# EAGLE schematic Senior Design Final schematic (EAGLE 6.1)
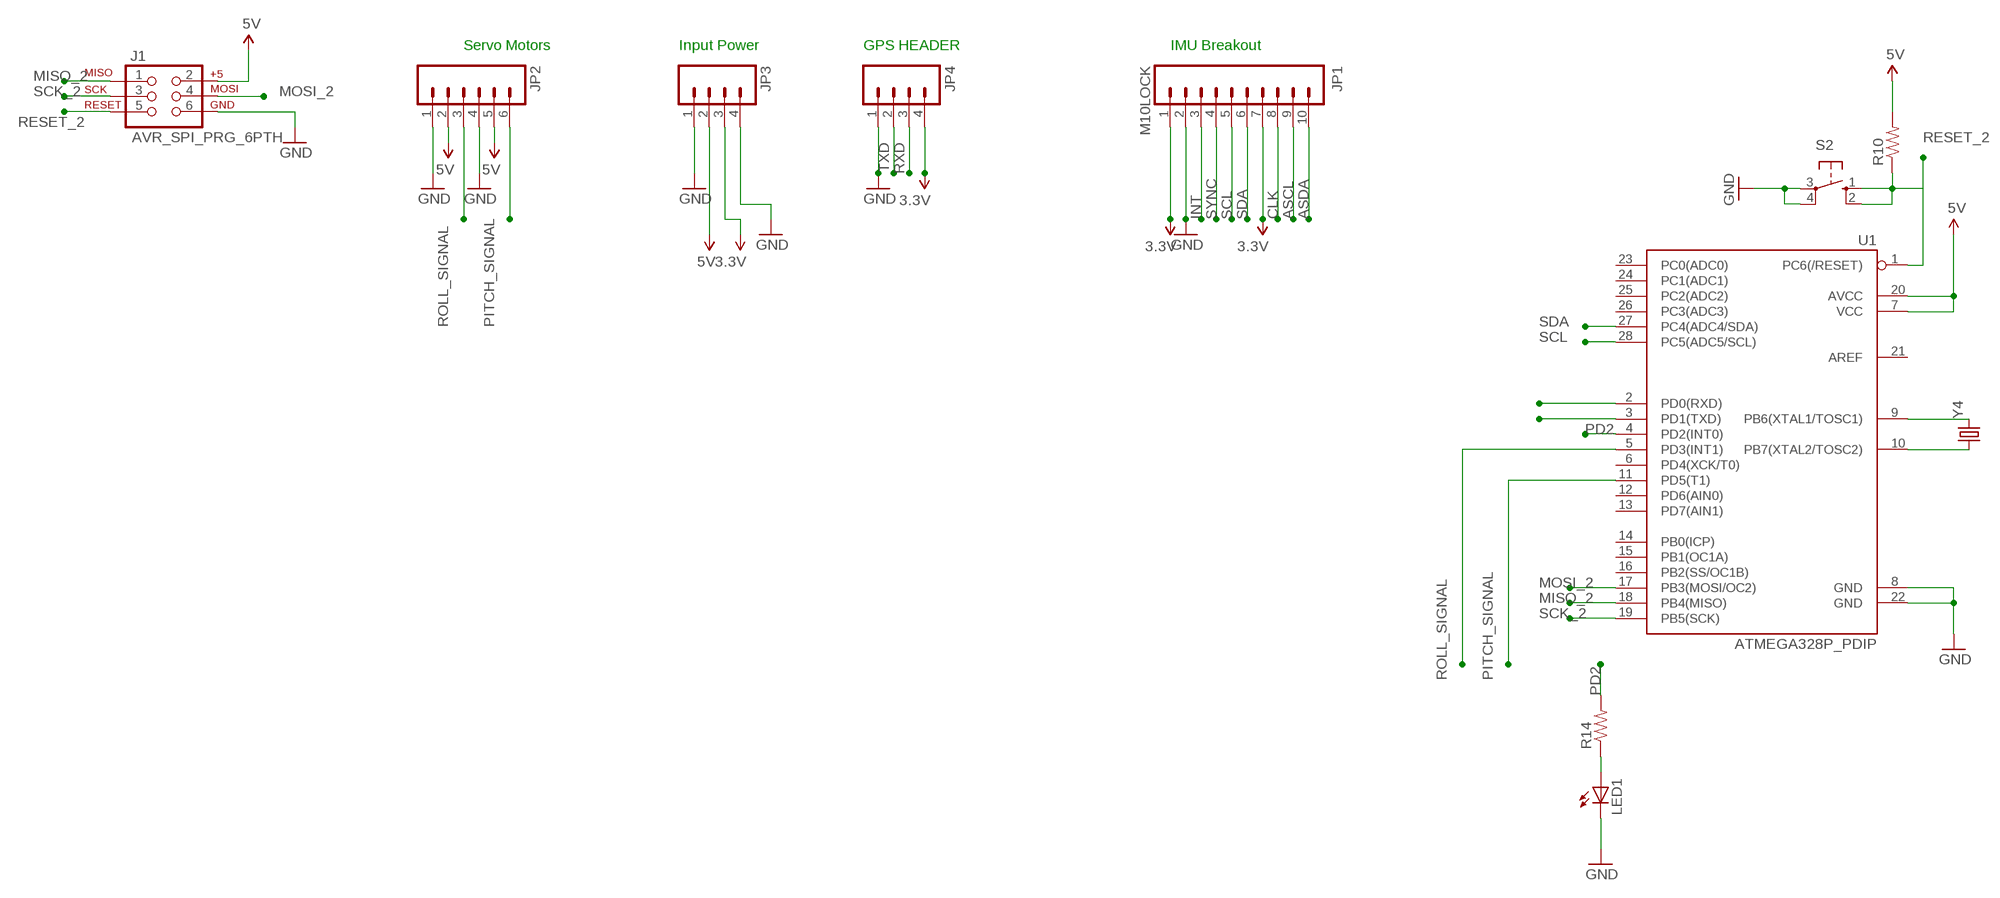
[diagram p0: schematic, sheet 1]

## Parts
J1  AVR_SPI_PRG_6PTH  [2X3]
JP1  M10LOCK  [1X10_LOCK]
JP2  M06LOCK  [1X06_LOCK]
JP3  M04LOCK  [1X04_LOCK]
JP4  M04LOCK  [1X04_LOCK]
LED1  LED5MM  [LED5MM]
R10  R-US_0207/10  [0207/10]
R14  R-US_0207/10  [0207/10]
S2  40-XX  [B3F-40XX]
U1  ATMEGA328P_PDIP  [DIL28-3]
Y4  CRYSTALHC49US  [HC49US]

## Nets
3.3V: JP1.1 JP1.7 JP3.3 JP4.4
5V: J1.2 JP2.2 JP2.5 JP3.2 R10.2 U1.7(VCC) U1.20(AVCC)
ASCL: JP1.9
ASDA: JP1.10
CLK: JP1.8
GND: J1.6 JP1.2 JP2.1 JP2.4 JP3.1 JP3.4 JP4.1 LED1.K(C) S2.3(P) S2.4(P1) U1.8(GND) U1.22(GND)
INT: JP1.3
MISO_2: J1.1 U1.18(PB4(MISO))
MOSI_2: J1.4 U1.17(PB3(MOSI/OC2))
N$18: U1.9(PB6(XTAL1/TOSC1)) Y4.2
N$19: U1.10(PB7(XTAL2/TOSC2)) Y4.1
N$25: LED1.A R14.1
PD2: R14.2 U1.4(PD2(INT0))
PITCH_SIGNAL: JP2.6 U1.11(PD5(T1))
RESET_2: J1.5 R10.1 S2.1(S) S2.2(S1) U1.1(PC6(/RESET))
ROLL_SIGNAL: JP2.3 U1.5(PD3(INT1))
RXD: JP4.3 U1.2(PD0(RXD))
SCK_2: J1.3 U1.19(PB5(SCK))
SCL: JP1.5 U1.28(PC5(ADC5/SCL))
SDA: JP1.6 U1.27(PC4(ADC4/SDA))
SYNC: JP1.4
TXD: JP4.2 U1.3(PD1(TXD))
Unconnected: U1.6(PD4(XCK/T0)) U1.12(PD6(AIN0)) U1.13(PD7(AIN1)) U1.14(PB0(ICP)) U1.15(PB1(OC1A)) U1.16(PB2(SS/OC1B)) U1.21(AREF) U1.23(PC0(ADC0)) U1.24(PC1(ADC1)) U1.25(PC2(ADC2)) U1.26(PC3(ADC3))

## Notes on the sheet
- Servo Motors | Input Power | GPS HEADER | IMU Breakout

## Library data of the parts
J1 = SparkFun-Connectors:AVR_SPI_PRG_6: AVR ISP 6 Pin This is the reduced ISP connector for AVR programming. Common on Arduino. This footprint will take up less PCB space and can be used with a 10-pin to 6-pin adapter such as SKU: BOB-08508
JP1 = SparkFun-Connectors:M10: Header 10 Standard 10-pin 0.1" header. Use with straight break away headers (SKU : PRT-00116), right angle break away headers (PRT-00553), swiss pins (PRT-00743), machine pins (PRT-00117), and female headers (PRT-00115).
JP2 = SparkFun-Connectors:M06: Header 6 Standard 6-pin 0.1" header. Use with straight break away headers (SKU : PRT-00116), right angle break away headers (PRT-00553), swiss pins (PRT-00743), machine pins (PRT-00117), and female headers (PRT-00115). Molex polarized connector foot print use with SKU : PRT-08094 with associated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
JP3 JP4 = SparkFun-Connectors:M04: Header 4 Standard 4-pin 0.1" header. Use with straight break away headers (SKU : PRT-00116), right angle break away headers (PRT-00553), swiss pins (PRT-00743), machine pins (PRT-00117), and female headers (PRT-00115). Molex polarized connector foot print use with SKU : PRT-08231 with associated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
LED1 = SparkFun-LED:LED: LEDs
R10 R14 = rcl:R-US_: RESISTOR, American symbol
S2 = switch-omron:40-XX: OMRON SWITCH; MF: OMRON COMPONENTS USA; MPN: B3F-4000; OC_FARNELL: 176434; OC_NEWARK: 36K3105
U1 = SparkFun-DigitalIC:ATMEGA328P_PDIP: uC used in the Arduino 32kb flash, 1k EEPROM, 2k SRAM This is the through-hole version of this chip.
Y4 = SparkFun-FreqCtrl:CRYSTAL: Various standard crystals. Proven footprints. Spark Fun Electronics SKU : COM-00534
